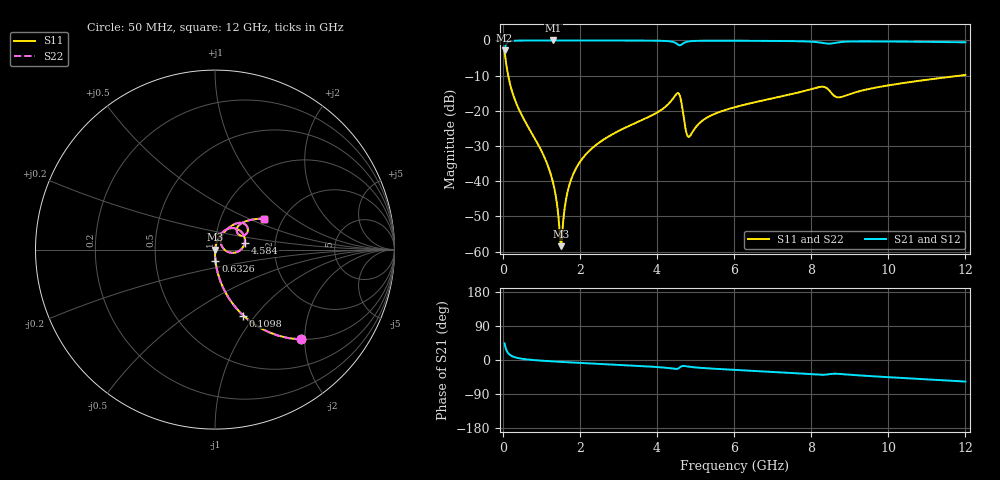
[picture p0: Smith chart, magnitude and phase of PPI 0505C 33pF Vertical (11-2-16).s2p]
# GHz S MA R 50
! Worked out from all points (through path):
!   1601 points, 50 MHz to 12 GHz, reference 50 ohm
!   highest |S21| = -0.01 dB at 1.312 GHz (marker M1); lowest = -2.8 dB at 50 MHz (marker M2)
!   group delay of S21, straight-line fit = 14 ps
!   lowest |S11| = -58.4 dB at 1.514 GHz (marker M3), VSWR 1.00, Z = 50.1 - j0.0043 ohm
!   |S11| at or under -10 dB: 143.1 MHz to 11.86 GHz (11.71 GHz wide, 195 % of centre)
!   |S22| runs from -58.4 to -3.2 dB; largest |S21 - S12| = 0
!   S11 on the Smith chart (normalised r, x): 50 MHz: 1.00, -1.92; 109.8 MHz: 1.00, -0.87; 632.6 MHz: 1.00, -0.13; 4.584 GHz: 1.39, +0.11; 12 GHz: 1.61, +0.62
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0.05  0.6929 -46.3  0.7208 43.7  0.7208 43.7  0.6929 -46.3
0.10975  0.3996 -66.8  0.9163 23.2  0.9163 23.2  0.3996 -66.8
0.2964688  0.1542 -81.9  0.9874 7.9  0.9874 7.9  0.1542 -81.9
0.6325625  0.06279 -87.7  0.9972 1.5  0.9972 1.5  0.06279 -87.7
1.080688  0.022 -89.6  0.9987 -2.3  0.9987 -2.3  0.022 -89.6
1.312219  0.009252 -86.9  0.9988 -3.8  0.9988 -3.8  0.009252 -86.9
1.476531  0.001952 -57.6  0.9987 -4.8  0.9987 -4.8  0.001952 -57.6
1.513875  0.001196 -2.1  0.9987 -5.0  0.9987 -5.0  0.001196 -2.1
1.723  0.008611 75.3  0.9986 -6.2  0.9986 -6.2  0.008611 75.3
2.044156  0.0202 78.2  0.9983 -7.9  0.9983 -7.9  0.0202 78.2
2.671531  0.04082 76.6  0.9973 -11.1  0.9973 -11.1  0.04082 76.6
4.038312  0.09705 67.9  0.9894 -18.8  0.9894 -18.8  0.09705 67.9
4.583531  0.1698 12.9  0.8534 -20.3  0.8534 -20.3  0.1698 12.9
4.755312  0.05141 1.0  0.9505 -16.4  0.9505 -16.4  0.05141 1.0
4.83  0.04274 29.1  0.9699 -17.6  0.9699 -17.6  0.04274 29.1
5.270656  0.07844 63.1  0.9895 -21.7  0.9895 -21.7  0.07844 63.1
6.025  0.1128 61.8  0.9891 -26.1  0.9891 -26.1  0.1128 61.8
8.019156  0.2049 46.8  0.9589 -37.7  0.9589 -37.7  0.2049 46.8
8.340312  0.2183 33.6  0.9119 -38.9  0.9119 -38.9  0.2183 33.6
8.721219  0.1551 36.2  0.9426 -36.6  0.9426 -36.6  0.1551 36.2
10.01331  0.2304 42.9  0.9656 -45.4  0.9656 -45.4  0.2304 42.9
12  0.3231 32.2  0.9403 -56.9  0.9403 -56.9  0.3231 32.2
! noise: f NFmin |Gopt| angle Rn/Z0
0.05  0.0003882  0.8647  0.7505  0.0006161
1.372  0.003998  0.675  4.55  0.002369
2.701  0.006829  0.6353  8.632  0.003506
4.031  0.01497  0.7373  12.95  0.01125
5.36  0.01833  0.7195  17.24  0.01265
6.682  0.0169  0.641  20.91  0.008618
8.012  0.03929  0.7987  25.59  0.03847
9.341  0.03255  0.7303  29.44  0.02253
10.67  0.0252  0.6304  32.37  0.01185
12  0.02585  0.6069  35.51  0.0111
